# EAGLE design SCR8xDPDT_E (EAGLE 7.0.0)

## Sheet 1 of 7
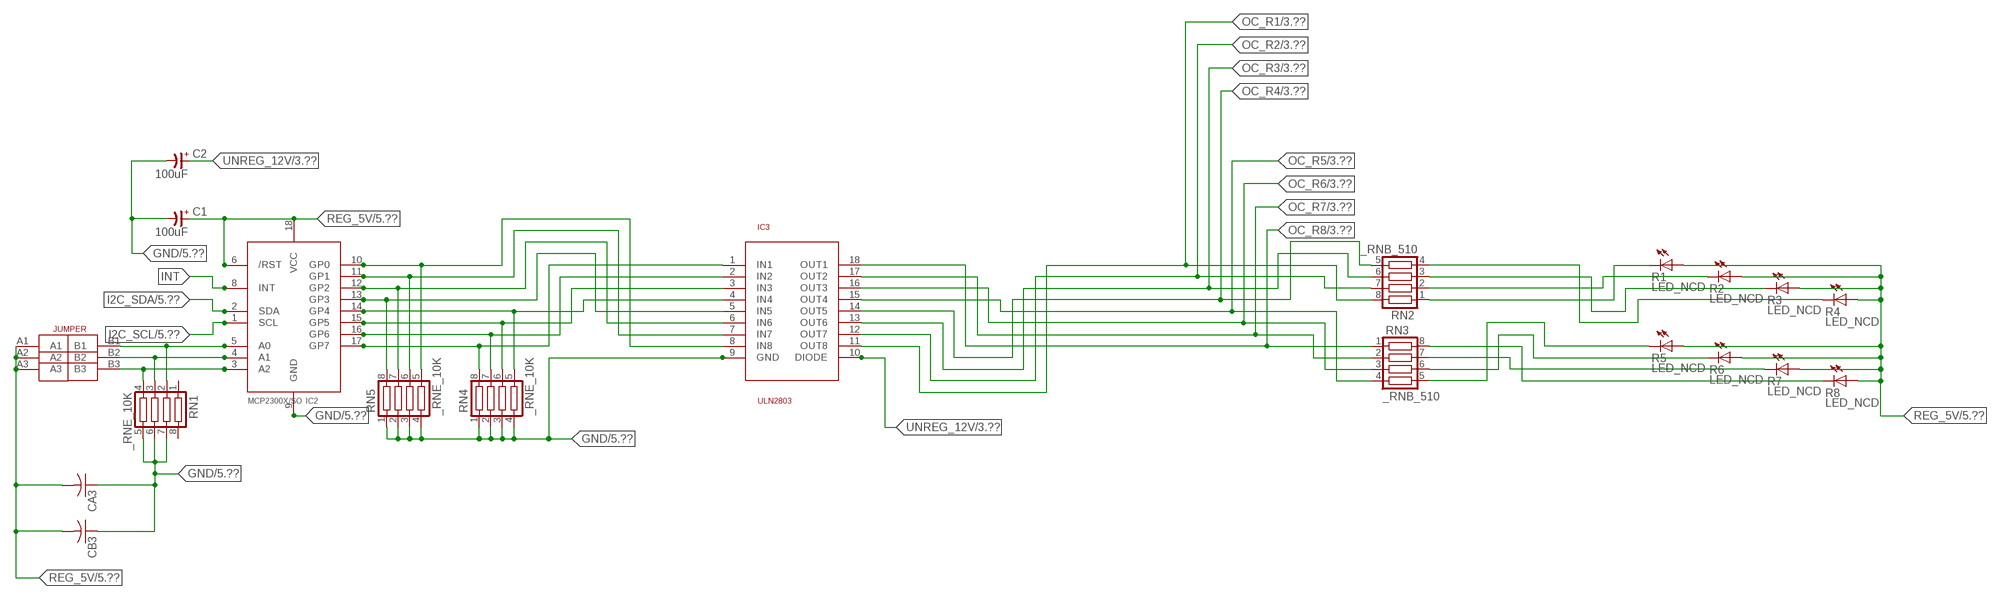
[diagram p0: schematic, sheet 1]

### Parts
C1  100uF  CP-E-025X060  [E-025X060]
C2  100uF  CP-E-025X060  [E-025X060]
CA3  CC1206KRX7R9BB104C1206K  [CC1206KRX7R9BB104]
CB3  TMK316F106ZL-TC1206K  [TMK316F106ZL-T]
IC2  MCP2300X/SO  [SO18W]
IC3  ULN2803  [SO18L]
R1  LED_NCD  [CHIPLED_0603]
R2  LED_NCD  [CHIPLED_0603]
R3  LED_NCD  [CHIPLED_0603]
R4  LED_NCD  [CHIPLED_0603]
R5  LED_NCD  [CHIPLED_0603]
R6  LED_NCD  [CHIPLED_0603]
R7  LED_NCD  [CHIPLED_0603]
R8  LED_NCD  [CHIPLED_0603]
RN1  _RNE_10K  [RNE]
RN2  _RNB_510  [RNB]
RN3  _RNB_510  [RNB]
RN4  _RNE_10K  [RNE]
RN5  _RNE_10K  [RNE]
U$18  JUMPER_3X2  [JUMPER_3X2]

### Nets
GND: C1.- C2.- CA3.1 CB3.1 IC2.9(GND) IC3.9(GND) RN1.5 RN1.6 RN1.7 RN4.1 RN4.2 RN4.3 RN4.4 RN5.1 RN5.2 RN5.3 RN5.4 ; also sheet 5,7
GP4: IC2.14(GP4) IC3.4(IN4) RN4.5
GP6: IC2.16(GP6) IC3.2(IN2) RN4.7
I2C_SCL: IC2.1(SCL) ; also sheet 5
I2C_SDA: IC2.2(SDA) ; also sheet 5
INT: IC2.8(INT)
N$6: IC2.5(A0) RN1.2 U$18.B1
N$7: IC2.4(A1) RN1.3 U$18.B2
N$8: IC2.3(A2) RN1.4 U$18.B3
N$20: R1.C RN2.1
N$21: IC2.12(GP2) IC3.6(IN6) RN5.7
N$22: IC2.11(GP1) IC3.7(IN7) RN5.6
N$23: IC2.10(GP0) IC3.8(IN8) RN5.5
N$29: R2.C RN2.2
N$30: R3.C RN2.3
N$31: R4.C RN2.4
N$32: R8.C RN3.8
N$81: R7.C RN3.7
N$82: R6.C RN3.6
N$83: R5.C RN3.5
N$89: IC2.13(GP3) IC3.5(IN5) RN5.8
N$93: IC2.15(GP5) IC3.3(IN3) RN4.6
N$94: IC2.17(GP7) IC3.1(IN1) RN4.8
OC_R1: IC3.11(OUT8) RN2.8 ; also sheet 3
OC_R2: IC3.12(OUT7) RN2.7 ; also sheet 3
OC_R3: IC3.13(OUT6) RN2.6 ; also sheet 3
OC_R4: IC3.14(OUT5) RN2.5 ; also sheet 3
OC_R5: IC3.15(OUT4) RN3.4 ; also sheet 3
OC_R6: IC3.16(OUT3) RN3.3 ; also sheet 3
OC_R7: IC3.17(OUT2) RN3.2 ; also sheet 3
OC_R8: IC3.18(OUT1) RN3.1 ; also sheet 3
REG_5V: C1.+ CA3.2 CB3.2 IC2.6(/RST) IC2.18(VCC) R1.A R2.A R3.A R4.A R5.A R6.A R7.A R8.A U$18.A1 U$18.A2 U$18.A3 ; also sheet 5,7
UNREG_12V: C2.+ IC3.10(DIODE) ; also sheet 3,5
Unconnected: RN1.1 RN1.8

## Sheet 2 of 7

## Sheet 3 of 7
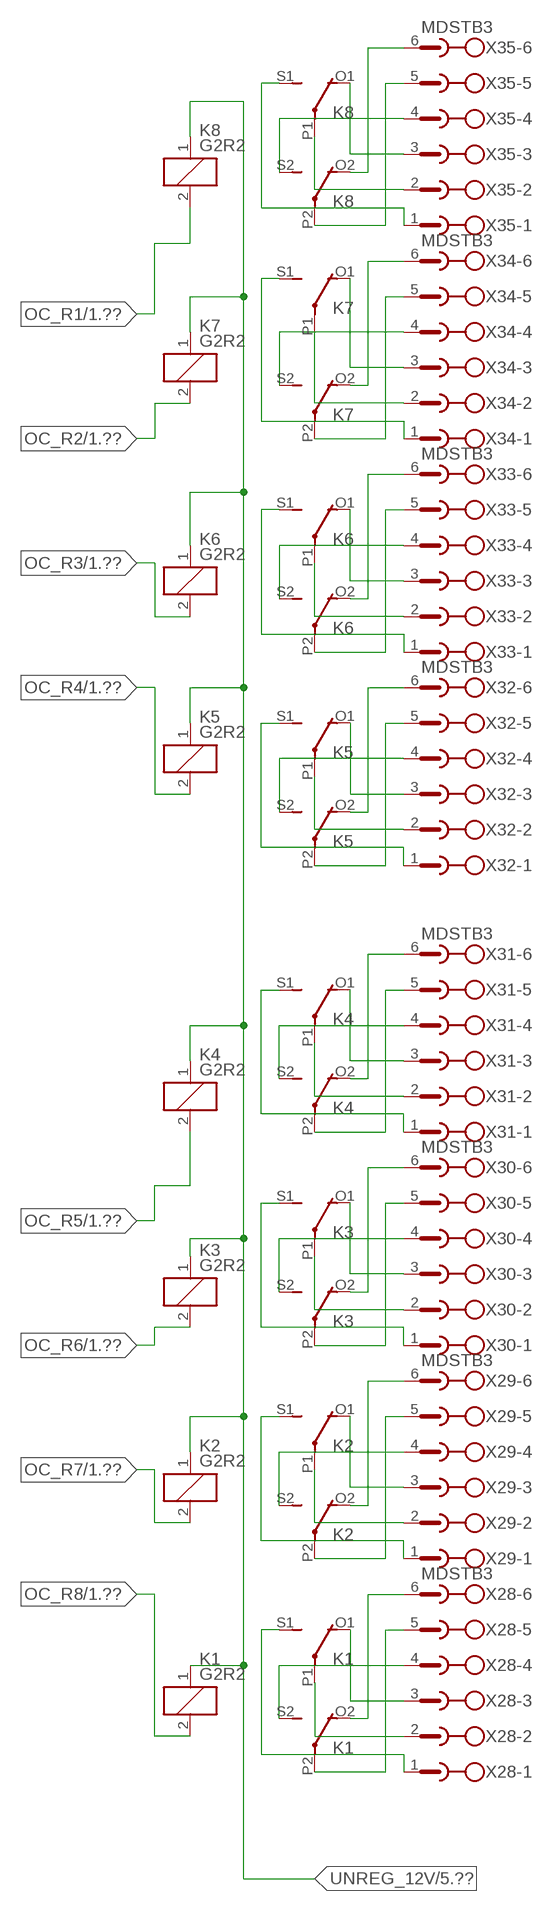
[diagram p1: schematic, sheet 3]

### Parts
K1  G2R2  [G2R2]
K2  G2R2  [G2R2]
K3  G2R2  [G2R2]
K4  G2R2  [G2R2]
K5  G2R2  [G2R2]
K6  G2R2  [G2R2]
K7  G2R2  [G2R2]
K8  G2R2  [G2R2]
X28  MDSTB3  [MDSTB3]
X29  MDSTB3  [MDSTB3]
X30  MDSTB3  [MDSTB3]
X31  MDSTB3  [MDSTB3]
X32  MDSTB3  [MDSTB3]
X33  MDSTB3  [MDSTB3]
X34  MDSTB3  [MDSTB3]
X35  MDSTB3  [MDSTB3]

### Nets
N$84: K1.P2(3:COM) X28.5
N$85: K1.O2(3:NC) X28.6
N$86: K1.S2(3:NO) X28.4
N$87: K1.P1(2:COM) X28.2
N$88: K1.O1(2:NC) X28.3
N$90: K1.S1(2:NO) X28.1
N$91: K2.P2(3:COM) X29.5
N$92: K2.O2(3:NC) X29.6
N$95: K2.S2(3:NO) X29.4
N$96: K2.S1(2:NO) X29.1
N$97: K2.P1(2:COM) X29.2
N$98: K2.O1(2:NC) X29.3
N$99: K3.P2(3:COM) X30.5
N$100: K3.O2(3:NC) X30.6
N$101: K4.P2(3:COM) X31.5
N$102: K4.O2(3:NC) X31.6
N$103: K3.S2(3:NO) X30.4
N$104: K4.S2(3:NO) X31.4
N$105: K3.O1(2:NC) X30.3
N$106: K4.O1(2:NC) X31.3
N$107: K4.P1(2:COM) X31.2
N$108: K3.P1(2:COM) X30.2
N$109: K3.S1(2:NO) X30.1
N$110: K4.S1(2:NO) X31.1
N$111: K5.O2(3:NC) X32.6
N$112: K5.P2(3:COM) X32.5
N$113: K5.S2(3:NO) X32.4
N$114: K5.P1(2:COM) X32.2
N$115: K5.S1(2:NO) X32.1
N$116: K5.O1(2:NC) X32.3
N$117: K6.P2(3:COM) X33.5
N$118: K6.O2(3:NC) X33.6
N$119: K6.P1(2:COM) X33.2
N$120: K6.S1(2:NO) X33.1
N$121: K7.P1(2:COM) X34.2
N$122: K8.P1(2:COM) X35.2
N$316: K8.P2(3:COM) X35.5
N$317: K8.O2(3:NC) X35.6
N$318: K6.O1(2:NC) X33.3
N$319: K8.O1(2:NC) X35.3
N$320: K7.O1(2:NC) X34.3
N$321: K7.O2(3:NC) X34.6
N$322: K7.P2(3:COM) X34.5
N$323: K6.S2(3:NO) X33.4
N$324: K7.S2(3:NO) X34.4
N$325: K7.S1(2:NO) X34.1
N$326: K8.S1(2:NO) X35.1
N$327: K8.S2(3:NO) X35.4
OC_R1: K8.2(1:C2) ; also sheet 1
OC_R2: K7.2(1:C2) ; also sheet 1
OC_R3: K6.2(1:C2) ; also sheet 1
OC_R4: K5.2(1:C2) ; also sheet 1
OC_R5: K4.2(1:C2) ; also sheet 1
OC_R6: K3.2(1:C2) ; also sheet 1
OC_R7: K2.2(1:C2) ; also sheet 1
OC_R8: K1.2(1:C2) ; also sheet 1
UNREG_12V: K1.1(1:C1) K2.1(1:C1) K3.1(1:C1) K4.1(1:C1) K5.1(1:C1) K6.1(1:C1) K7.1(1:C1) K8.1(1:C1) ; also sheet 1,5

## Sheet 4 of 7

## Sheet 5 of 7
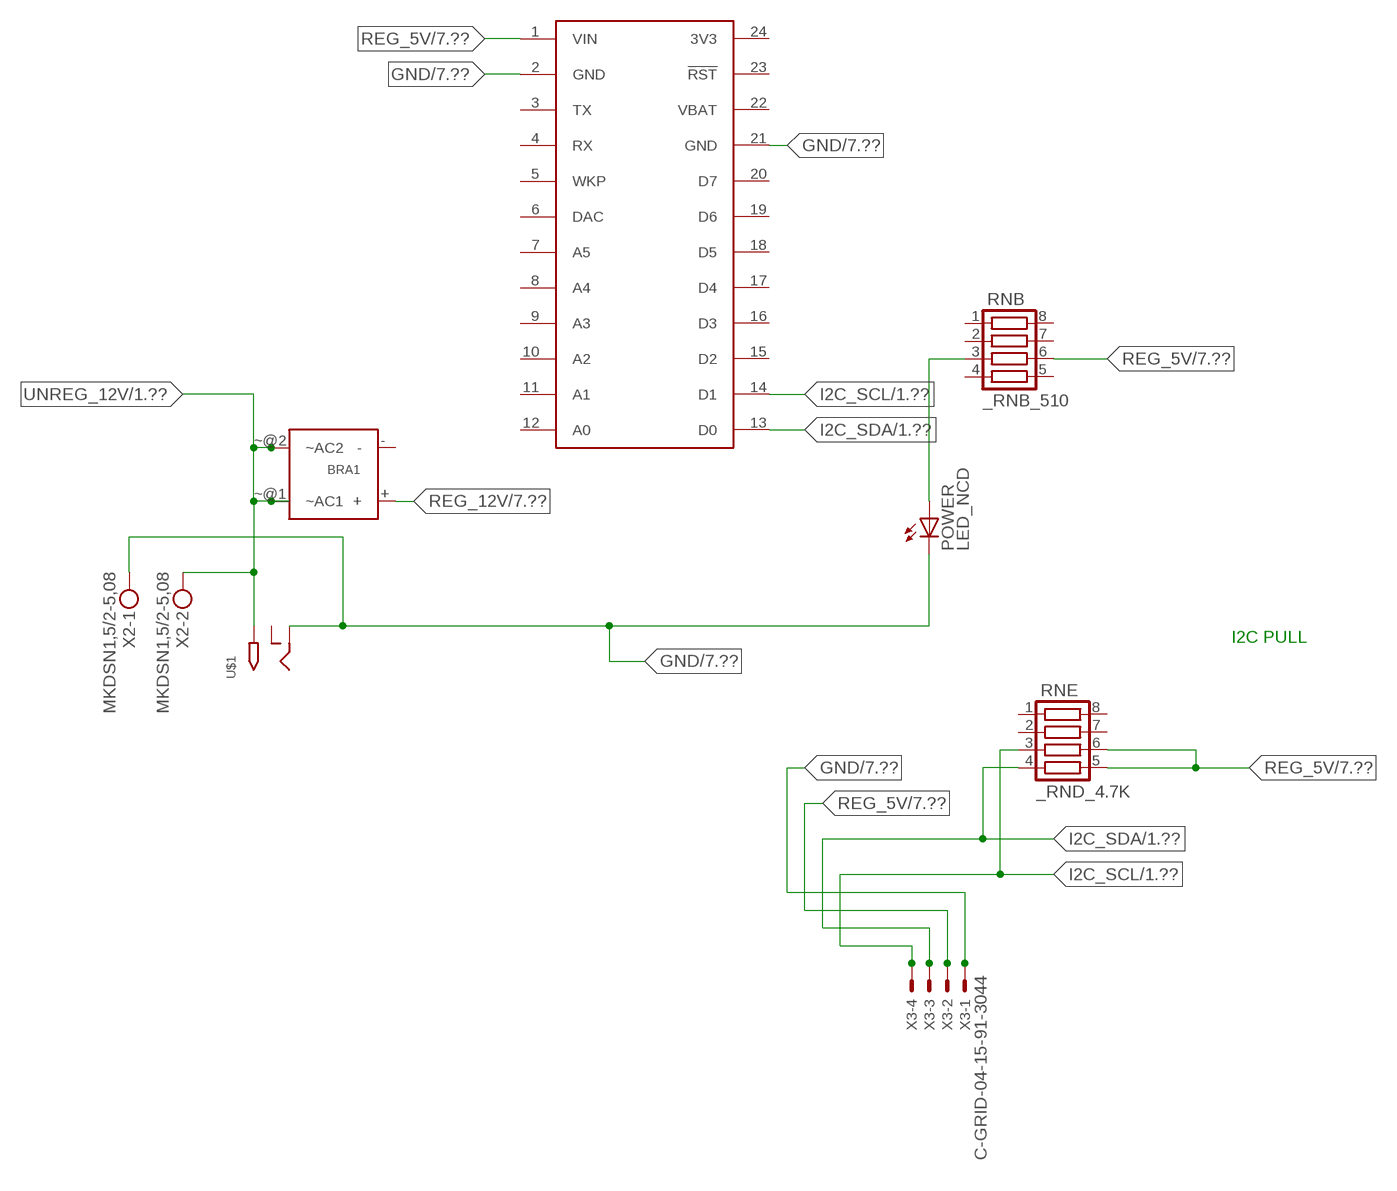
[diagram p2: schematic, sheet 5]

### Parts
BRA1  MB2S_  [MB2S]
POWER  LED_NCD  [CHIPLED_0603]
RNB  _RNB_510  [RNB]
RNE  _RND_4.7K  [RND]
S1  SPARK_CORECORE  [SPARK_CORE]
U$1  2.1MMJACK  [PJ-102A]
X2  MKDSN1,5/2-5,08  [MKDSN1,5/2-5,08]
X3  C-GRID-04-15-91-3044  [15-91-04]

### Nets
GND: POWER.C S1.2(GND) S1.21(GND) U$1.RING X2.1 X3.1 ; also sheet 1,7
I2C_SCL: RNE.3 S1.14(D1) X3.4 ; also sheet 1
I2C_SDA: RNE.4 S1.13(D0) X3.3 ; also sheet 1
N$2: POWER.A RNB.3
REG_5V: RNB.6 RNE.5 RNE.6 S1.1(VIN) X3.2 ; also sheet 1,7
REG_12V: BRA1.+ ; also sheet 7
UNREG_12V: BRA1.~@1(~AC1) BRA1.~@2(~AC2) U$1.TIP X2.2 ; also sheet 1,3
Unconnected: BRA1.- RNB.1 RNB.2 RNB.4 RNB.5 RNB.7 RNB.8 RNE.1 RNE.2 RNE.7 RNE.8 S1.3(TX) S1.4(RX) S1.5(WKP) S1.6(DAC) S1.7(A5) S1.8(A4) S1.9(A3) S1.10(A2) S1.11(A1) S1.12(A0) S1.15(D2) S1.16(D3) S1.17(D4) S1.18(D5) S1.19(D6) S1.20(D7) S1.23(!RST) U$1.RING_SW

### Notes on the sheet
- I2C PULL

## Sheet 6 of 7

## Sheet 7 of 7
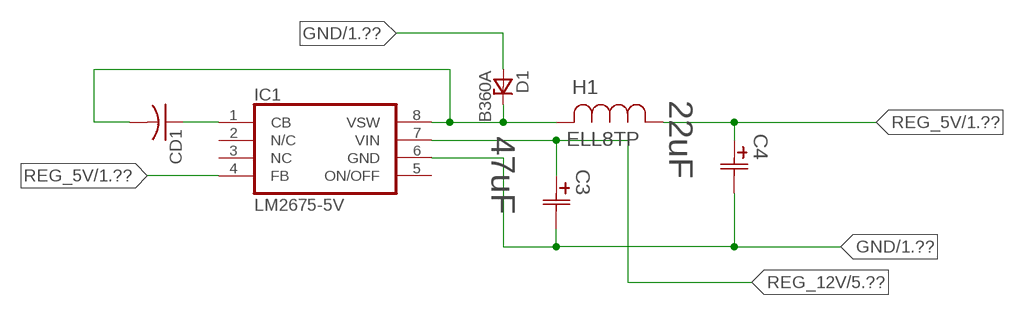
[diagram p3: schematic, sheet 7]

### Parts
C3  47uF  490-5463-6-NDCAP  [C2917(7343)-Y]
C4  22uF  490-5463-6-NDCAP  [C2917(7343)-Y]
CD1  _CD_10NF_50VC1206K  [_CD_10NF_50V]
D1  B360A  [DO214AC_ZENER]
H1  ELL8TP  [IND_ELL8TP]
IC1  LM2675-5V  LM2675  [SO-8]

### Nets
GND: C3.2(C2) C4.2(C2) D1.A IC1.6(GND) ; also sheet 1,5
N$1: CD1.2 D1.C H1.2 IC1.8(VSW)
N$3: CD1.1 IC1.1(CB)
REG_5V: C4.1(C1) H1.1 IC1.4(FB) ; also sheet 1,5
REG_12V: C3.1(C1) IC1.7(VIN) ; also sheet 5
Unconnected: IC1.2(N/C) IC1.5(ON/OFF)

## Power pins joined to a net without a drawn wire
3V3: S1.24(3V3)
NC: IC1.3(NC)
VBAT: S1.22(VBAT)

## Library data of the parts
BRA1 = NCD_ULTIMATE_LIBRARY:MB2S: Bridge Rectifier BRA MB2S 200V 500ma Digikey MB2S-TPMSTR-ND/MB2S-TP
C1 C2 = NCD_ULTIMATE_LIBRARY:CP-: Capacitors All Kinds POLARIZED CAP
C3 C4 = NCD_ULTIMATE_bhaskar:490-5463-6-ND: NCD CAP
CA3 = NCD_ULTIMATE_LIBRARY:CC1206KRX7R9BB104: Capacitor CA .1uF 50V SMT C1206K CC1206KRX7R9BB104
CB3 = NCD_ULTIMATE_LIBRARY:TMK316F106ZL-T: Capacitor CB 10uF SMT 1206 TMK316F106ZL-T
CD1 = NCD_ULTIMATE_LIBRARY:_CD_10NF_50V: Capacitor 10nF SMT
D1 = NCD_ULTIMATE_bhaskar:B360A: NCD DIODE B350A/B360A
H1 = NCD_ULTIMATE_bhaskar:ELL8TP: NCD coil
IC1 = NCD_ULTIMATE_bhaskar:LM2675: LM2675 NCD http://www.ti.com/lit/ds/symlink/lm2675.pdf
IC2 = NCD_ULTIMATE_LIBRARY:MCP2300X: Semiconductor Port Expander I/O 8-Bit I2C MCP23008 Inexpensive i2c i/o expander - 8 general purpose i/o pins with optional pullups
IC3 = NCD_ULTIMATE_LIBRARY:ULN2803: Semiconductor 8 O.C. N-Channel Transistor Driver Digikey ULN2803AFWGCELTR-ND/ULN2803AFWG,C,EL
K1-K8 = NCD_ULTIMATE_LIBRARY:G2R2: RELAY 2 x switch, Omron
POWER = NCD_ULTIMATE_bhaskar:LED_NCD
R1-R8 = NCD_ULTIMATE_LIBRARY:LED_NCD: LED Digikey 754-1132-2-ND/APT2012SRCPRV
RN1 RN4 RN5 = NCD_ULTIMATE_LIBRARY:_RNE_10K: Resistor Array RNE SMT 10K x 4 Single Resistor Source: http://www.ctscorp.com/components/Datasheets/CTSChipArrayDs.pdf Digikey 742C083103JPTR-ND/742C083103JP; OC_FARNELL: unknown; OC_NEWARK: unknown
RN2 RN3 RNB = NCD_ULTIMATE_LIBRARY:_RNB_510: Resistor Array RNB SMT 510 x 4 Single Resistor Source: http://www.ctscorp.com/components/Datasheets/CTSChipArrayDs.pdf Digikey 742C083511JPTR-ND/ 742C083511JP; OC_FARNELL: unknown; OC_NEWARK: unknown
RNE = NCD_ULTIMATE_LIBRARY:_RND_4.7K: Resistor Array RND SMT 4.7K x 4 Single Resistor Source: http://www.ctscorp.com/components/Datasheets/CTSChipArrayDs.pdf Digikey 742C083472JPTR-ND/742C083472JP; OC_FARNELL: unknown; OC_NEWARK: unknown
S1 = Spark:SPARK_CORE
U$1 = NCD_ULTIMATE_CONNECTORS:2.1MMJACK: 2.1mm x 5.5mm DC jack with internal switch. Digikey part #PJ-102A, 4UCON part #05537 By microbuilder.eu
U$18 = NCD_ULTIMATE_CONNECTORS:JUMPER_3X2
X2 = NCD_ULTIMATE_CONNECTORS:MKDSN1,5/2-5,08: MKDSN 1,5/ 2-5,08 Printklemme
X3 = NCD_ULTIMATE_CONNECTORS:C-GRID-04: CONNECTOR 4-Pos I2C wire to board 2.54 mm (0.100") pitch header Digikey WM1342-ND/0015912045; OC_FARNELL: unknown; OC_NEWARK: unknown
X28-X35 = NCD_ULTIMATE_LIBRARY:MDSTB3: PHOENIX

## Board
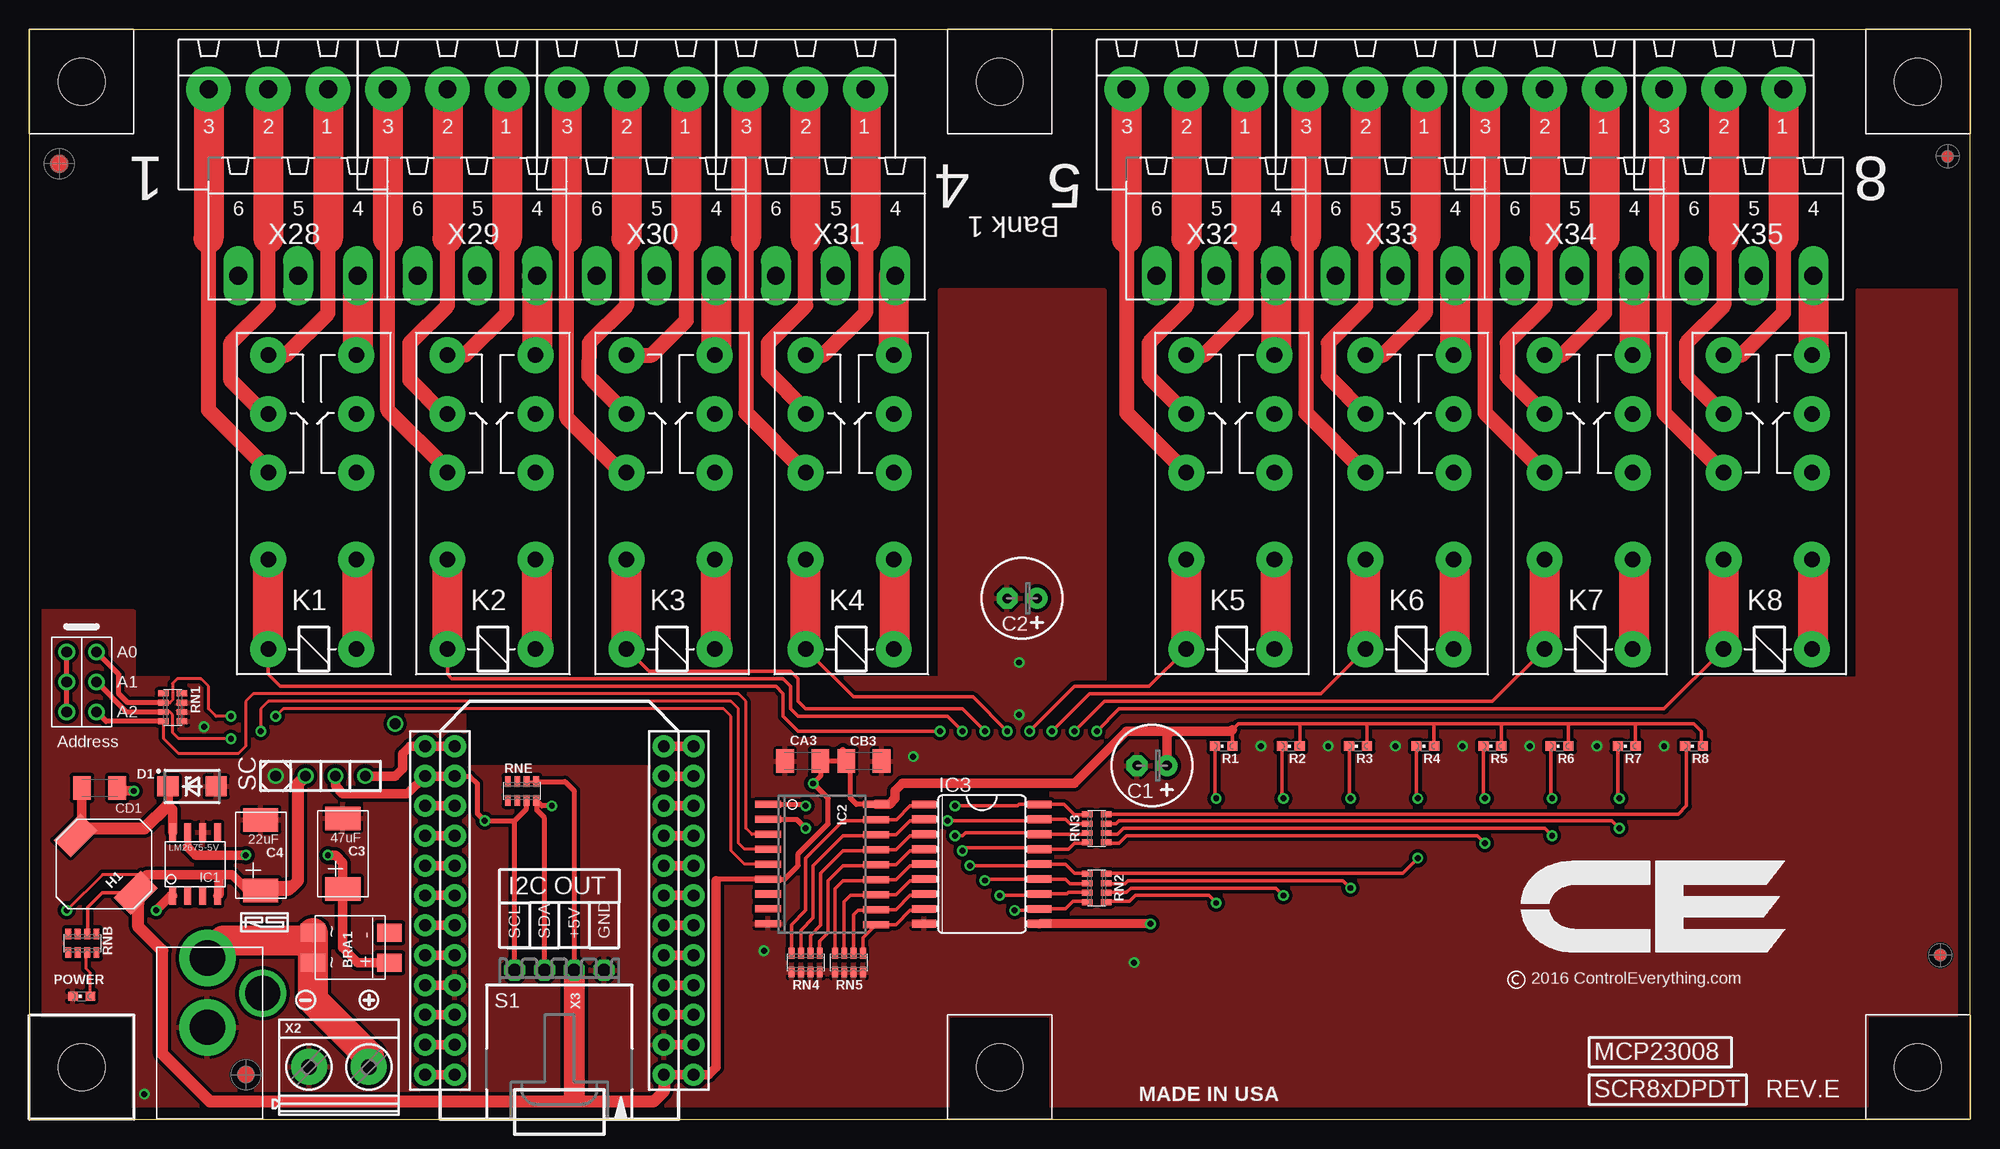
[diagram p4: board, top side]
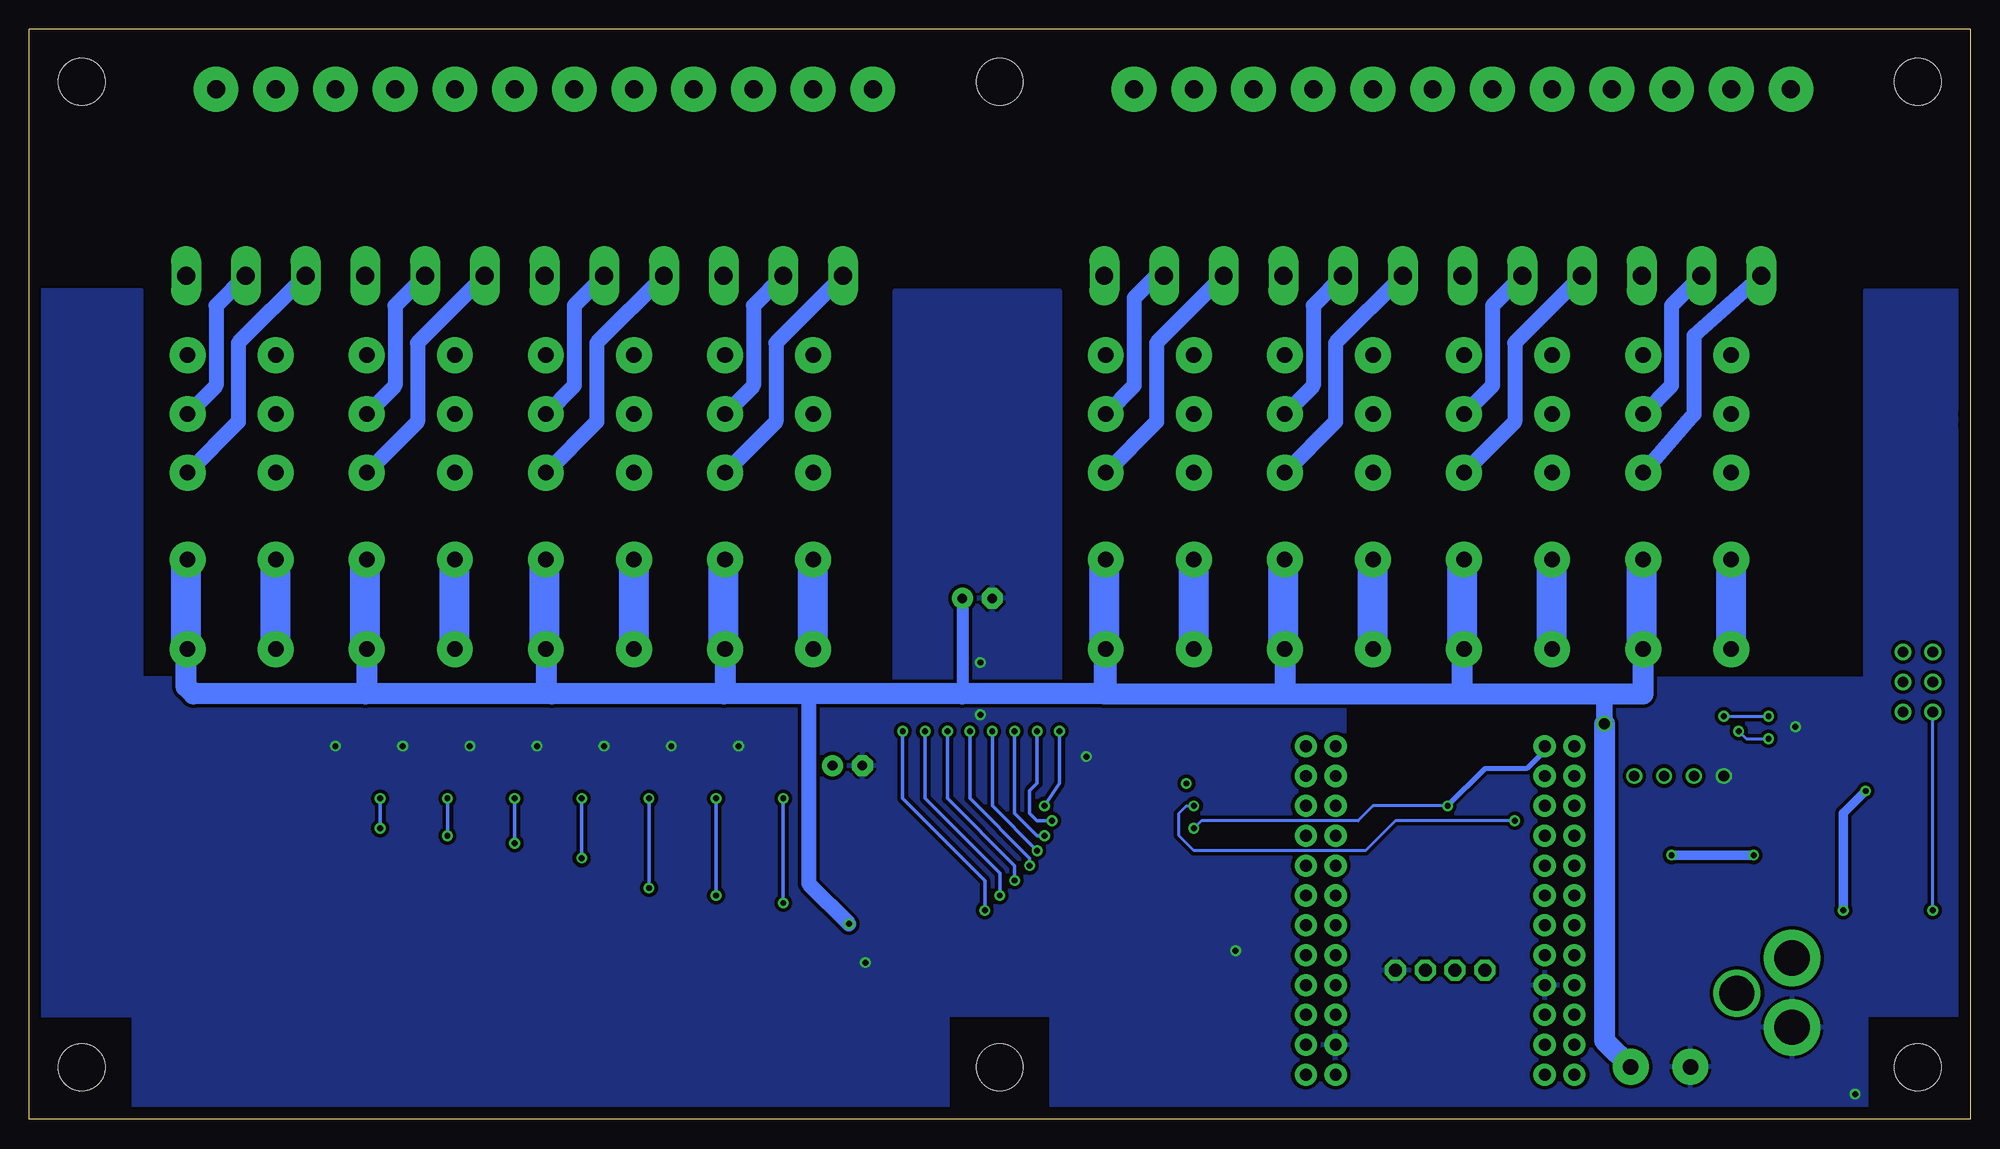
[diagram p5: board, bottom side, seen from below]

Size 165.1 x 92.71 mm. Coordinates in mm from the lower left corner, seen from the top.
Outline: 81.28,0 82.53,0
Outline: 0,59.99 0,59.05
Outline: 0,59.05 0,0 81.28,0
Outline: 81.28,0 165.1,0 165.1,92.71 0,92.71 0,59.05
Copper layers (1*16): Top 0.035mm / dielectric 1.5mm / Bottom 0.035mm
Design rules "default": minimum track width 10mil, minimum drill 24mil, track to track 8mil, track to pad 8mil, pad to pad 8mil, via to via 8mil, smd to smd 8mil, copper to edge 40mil, drill to drill 8mil, minimum pad ring 10mil, minimum via ring 8mil, stop-mask expansion 4mil, vias tented up to drill 0mil, thermal gap 10mil
Holes 3.96 mm at 4.45,4.45 4.45,4.45

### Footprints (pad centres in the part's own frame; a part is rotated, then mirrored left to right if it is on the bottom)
MB2S = smd 1.55 x 2.1: + 0,-6.5; - 2.54,-6.5; ~@1 0,0; ~@2 2.54,0
E-025X060 = drill 0.813 pad 1.778: + -1.27,0 | drill 0.813 pad 1.778 octagon: - 1.27,0
C2917(7343)-Y = smd 2 x 3: 1 -3,0; 2 3,0
CC1206KRX7R9BB104 = smd 1.5 x 2: 1 -1.5,0; 2 1.5,0
TMK316F106ZL-T = smd 1.5 x 2: 1 -1.5,0; 2 1.5,0
_CD_10NF_50V = smd 1.5 x 2: 1 -1.5,0; 2 1.5,0
DO214AC_ZENER = smd 1.8 x 1.7: A 2.05,0; C -2.05,0
IND_ELL8TP = smd 2.054 x 3.2 rotated 45: 1 -2.442,-2.696; 2 2.442,2.442
SO-8 = smd 0.6 x 1.55: 1 -1.905,-2.69; 2 -0.635,-2.69; 3 0.635,-2.69; 4 1.905,-2.69; 5 1.905,2.71; 6 0.635,2.71; 7 -0.635,2.71; 8 -1.905,2.71
SO18W = smd 0.6 x 2.2: 1 -4.445,-4.6; 2 -3.175,-4.6; 3 -1.905,-4.6; 4 -0.635,-4.6; 5 0.635,-4.6; 6 1.905,-4.6; 7 3.175,-4.6; 8 4.445,-4.6; 9 5.715,-4.6; 10 5.775,4.6; 11 4.505,4.6; 12 3.235,4.6; 13 1.965,4.6; 14 0.695,4.6; 15 -0.575,4.6; 16 -1.845,4.6; 17 -3.145,4.6; 18 -4.445,4.6
SO18L = smd 0.66 x 2.032: 1 -5.08,-4.902; 2 -3.81,-4.902; 3 -2.54,-4.902; 4 -1.27,-4.902; 5 0,-4.902; 6 1.27,-4.902; 7 2.54,-4.902; 8 3.81,-4.902; 9 5.08,-4.902; 10 5.08,4.902; 11 3.81,4.902; 12 2.54,4.902; 13 1.27,4.902; 14 0,4.902; 15 -1.27,4.902; 16 -2.54,4.902; 17 -3.81,4.902; 18 -5.08,4.902
G2R2 = drill 1.321 pad 3.048: 1 -2.54,-3.683; 2 -2.54,3.81; 3 5.08,-3.683; 4 5.08,3.81; O1 12.471,3.81; O2 12.471,-3.683; P1 17.45,3.81; P2 17.45,-3.683; S1 22.454,3.81; S2 22.454,-3.683
CHIPLED_0603 = smd 0.8 x 0.8: A 0,-0.75; C 0,0.75
CHIPLED_0603' = smd 0.8 x 0.876: A 0,-0.75; C 0,0.75
RNE = smd 0.5 x 0.9: 1 -1.2,-0.8; 2 -0.4,-0.8; 3 0.4,-0.8; 4 1.2,-0.8; 5 1.2,0.8; 6 0.4,0.8; 7 -0.4,0.8; 8 -1.2,0.8
RNB = smd 0.5 x 0.9: 1 -1.2,-0.8; 2 -0.4,-0.8; 3 0.4,-0.8; 4 1.2,-0.8; 5 1.2,0.8; 6 0.4,0.8; 7 -0.4,0.8; 8 -1.2,0.8
RND = smd 0.5 x 0.9: 1 -1.2,-0.8; 2 -0.4,-0.8; 3 0.4,-0.8; 4 1.2,-0.8; 5 1.2,0.8; 6 0.4,0.8; 7 -0.4,0.8; 8 -1.2,0.8
SPARK_CORE = drill 1.016 pad 1.88: 1 -8.89,13.97; 2 -8.89,11.43; 3 -8.89,8.89; 4 -8.89,6.35; 5 -8.89,3.81; 6 -8.89,1.27; 7 -8.89,-1.27; 8 -8.89,-3.81; 9 -8.89,-6.35; 10 -8.89,-8.89; 11 -8.89,-11.43; 12 -8.89,-13.97; 13 8.89,-13.97; 14 8.89,-11.43; 15 8.89,-8.89; 16 8.89,-6.35; 17 8.89,-3.81; 18 8.89,-1.27; 19 8.89,1.27; 20 8.89,3.81; 21 8.89,6.35; 22 8.89,8.89; 23 8.89,11.43; 24 8.89,13.97; 25 -11.43,13.97; 26 -11.43,11.43; 27 -11.43,8.89; 28 -11.43,6.35; 29 -11.43,3.81; 30 -11.43,1.27; 31 -11.43,-1.27; 32 -11.43,-3.81; 33 -11.43,-6.35; 34 -11.43,-8.89; 35 -11.43,-11.43; 36 -11.43,-13.97; 37 11.43,13.97; 38 11.43,11.43; 39 11.43,8.89; 40 11.43,6.35; 41 11.43,3.81; 42 11.43,1.27; 43 11.43,-1.27; 44 11.43,-3.81; 45 11.43,-6.35; 46 11.43,-8.89; 47 11.43,-11.43; 48 11.43,-13.97
PJ-102A = drill 3 pad 4.8: RING 0.1,-3.39; TIP 0.1,-9.29 | drill 3 pad 3.251: RING_SW -4.6,-6.29
PCB_MOUNTING_HOLE = hole 3.962: 4.445,4.445
JUMPER_3X2 = drill 0.9: A1 0,5.08; A2 0,2.54; A3 0,0; B1 2.54,5.08; B2 2.54,2.54; B3 2.54,0
MKDSN1,5/2-5,08 = drill 1.3 pad 3.048: 1 -2.561,0.025; 2 2.519,0.025
15-91-04 = drill 1.1 pad 1.778 octagon: 1 -3.81,-7.62; 2 -1.27,-7.62; 3 1.27,-7.62; 4 3.81,-7.62
MDSTB3 = drill 1.524 pad 3.81: 1 -3.81,-10.795; 2 1.27,-10.795; 3 6.35,-10.795 | drill 1.524 pad 2.54 long: 4 -6.35,5.08; 5 -1.27,5.08; 6 3.81,5.08

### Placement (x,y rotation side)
BRA1  24.13,13.34 90 top
C1  95.5,30.1 180 top
C2  84.45,44.32 180 top
C3  26.67,22.61 90 top
C4  19.68,22.48 90 top
CA3  65.79,30.48 0 top
CB3  70.99,30.48 180 top
CD1  5.97,28.19 180 top
D1  13.84,28.32 0 top
H1  6.35,21.72 90 top
IC1  14.1,21.72 0 top
IC2  67.44,22.35 270 top
IC3  81.03,21.72 270 top
K1  24.13,42.54 90 top
K2  39.37,42.54 90 top
K3  54.61,42.54 90 top
K4  69.85,42.54 90 top
K5  102.23,42.54 90 top
K6  117.47,42.54 90 top
K7  132.72,42.54 90 top
K8  147.96,42.54 90 top
POWER  4.45,10.48 90 top
R1  LED_NCD  [CHIPLED_0603']  101.6,31.75 90 top
R2  LED_NCD  [CHIPLED_0603']  107.31,31.75 90 top
R3  LED_NCD  [CHIPLED_0603']  113.03,31.75 90 top
R4  LED_NCD  [CHIPLED_0603']  118.75,31.75 90 top
R5  LED_NCD  [CHIPLED_0603']  124.46,31.75 90 top
R6  LED_NCD  [CHIPLED_0603']  130.18,31.75 90 top
R7  LED_NCD  [CHIPLED_0603']  135.89,31.75 90 top
R8  LED_NCD  [CHIPLED_0603']  141.6,31.75 90 top
RN1  12.19,35.05 270 top
RN2  90.81,19.69 90 top
RN3  90.81,24.77 270 top
RN4  66.04,13.34 0 top
RN5  69.72,13.34 0 top
RNB  4.51,14.99 0 top
RNE  41.91,27.94 0 top
S1  45.09,17.78 180 top
U$1  15.24,4.45 180 top
U$4  [VISION_REF10]  162.56,13.97 270 top
U$6  PCB_MOUNTING_HOLE  [PCB_MOUNTING_HOLE]  87,0 90 top
U$9  PCB_MOUNTING_HOLE  [PCB_MOUNTING_HOLE]  87,83.82 90 top
U$10  [VISION_REF15]  18.41,3.81 0 top
U$11  PCB_MOUNTING_HOLE  [PCB_MOUNTING_HOLE]  165.1,0 90 top
U$13  PCB_MOUNTING_HOLE  [PCB_MOUNTING_HOLE]  8.89,83.82 90 top
U$14  PCB_MOUNTING_HOLE  [PCB_MOUNTING_HOLE]  165.1,83.82 90 top
U$16  [VISION_REF10]  163.19,81.91 270 top
U$17  [VISION_REF15]  2.54,81.28 270 top
U$18  3.17,34.67 0 top
U$21  [ICON_USA]  94.36,1.52 0 top
U$22  [ICON_MINUS]  23.5,10.16 180 top
U$24  [ICON_PLUS]  28.89,10.16 90 top
X2  26.35,4.45 0 top
X3  45.09,5.08 180 top
X28  21.59,76.83 180 top
X29  36.83,76.83 180 top
X30  52.07,76.83 180 top
X31  67.31,76.83 180 top
X32  99.69,76.83 180 top
X33  114.94,76.83 180 top
X34  130.18,76.83 180 top
X35  145.41,76.83 180 top

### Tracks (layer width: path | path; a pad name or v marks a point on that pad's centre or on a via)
GND  (via drill 0.5, 0.9)
  other vias: 14.86,33.4 62.48,14.35 127.64,31.75 93.98,13.34 133.35,31.75 139.06,31.75 121.92,31.75 116.2,31.75 110.49,31.75 104.78,31.75 75.18,30.86 84.2,34.42 84.2,38.86 9.78,2.16 20.95,29.21
  pour Bottom (isolate 0.305): -1.27,8.89 8.89,8.89 8.89,0 78.11,0 78.11,8.89 91.44,8.89 91.44,70.48 77.47,70.48 77.47,37.46 8.89,37.46 8.89,70.48 -1.27,70.48
  pour Top (isolate 0.305): -3.17,8.89 8.89,8.89 8.89,0 78.11,0 78.11,8.89 91.44,8.89 91.44,70.48 77.47,70.48 77.47,37.46 8.89,37.46 8.89,43.18 -3.17,43.18
  pour Top (isolate 0.305): 87,37.46 155.57,37.46 155.57,70.48 168.28,70.48 168.28,8.89 156.21,8.89 156.21,0 87,0
  pour Bottom (isolate 0.305): 87,0 87,37.46 155.57,37.46 155.57,70.48 170.81,70.48 170.81,8.89 156.21,8.89 156.21,0
GP4
  Top 0.305: RN4.5 67.24,15.17 67.94,15.88 67.94,20.32 69.22,21.59 71.97,21.59 IC2.14 73.73,21.66 74.93,22.86 76,22.86 IC3.4
GP6
  Top 0.305: RN4.7 65.64,16.11 66.67,17.14 66.67,21.59 69.22,24.13 71.97,24.13 IC2.16 73.73,24.2 74.93,25.4 76,25.4 IC3.2
I2C_SCL  (via drill 0.5, 0.9)
  Top 0.406: IC2.1 65.91,26.8 v66.04,26.67 | X3.4 41.27,25.4 | 41.27,25.4 42.29,26.42 42.29,27.12 RNE.3 | S1.14 37.47,29.21 38.1,28.57 38.1,26.04 v38.73,25.4 41.27,25.4
  Top 0.813: v26.04,29.21 26.04,28.32 26.67,27.69 32.13,27.69 33.66,29.21
  Bottom 0.254: v38.73,25.4 48.9,25.4 51.44,22.86 66.04,22.86 67.31,24.13 67.31,26.04 66.67,26.67 v66.04,26.67
I2C_SDA  (via drill 0.5, 0.9)
  Top 0.406: IC2.2 65.28,25.53 v66.04,24.77 | X3.3 43.81,25.65 43.18,26.29 43.18,27.07 RNE.4 43.58,26.67 v44.45,26.67
  Top 0.813: v28.57,29.21 31.11,29.21 31.75,29.85 31.75,31.12 32.38,31.75 33.66,31.75
  Bottom 0.254: v44.45,26.67 50.8,26.67 52.07,25.4 65.41,25.4 v66.04,24.77
  Bottom 0.406: S1.13 36.2,31.37 37.72,29.85 41.27,29.85 v44.45,26.67
N$1
  Top 0.813: H1.2 3.88,24.77 | D1.C 11.79,26.78 12.19,26.38 IC1.8 | CD1.2 4.47,24.79 4.45,24.77
  Top 1.016: 3.88,24.77 4.45,24.77 9.78,24.77 11.79,26.78
N$2
  Top 0.254: POWER.A 5.2,12.46 4.83,12.83 4.83,14.1 RNB.3
  Top 0.406: 4.95,14.14 RNB.3
N$3  (via drill 0.5)
  Top 0.813: IC1.1 12.04,19.03 v10.79,17.78 | v8.89,27.94 7.72,27.94 CD1.1
  Bottom 0.813: v10.79,17.78 10.79,26.04 v8.89,27.94
N$6  (via drill 0.5)
  Top 0.254: IC2.5 60.83,21.72 59.69,22.86 59.69,34.29 59.05,34.92 21.59,34.92 v20.95,34.29 | v17.14,34.29 15.88,34.29 15.24,34.92 15.24,36.83 14.61,37.46 12.57,37.46 12.19,37.08 12.19,35.69 11.94,35.43 11.41,35.43 RN1.2
  Top 0.406: RN1.2 8.36,35.45 7.62,36.2 7.62,37.85 U$18.B1
  Bottom 0.254: v20.95,34.29 v17.14,34.29
N$7  (via drill 0.5)
  Top 0.254: IC2.4 60.83,22.99 60.33,23.5 60.33,34.92 59.69,35.56 20.32,35.56 19.68,34.92 v19.68,33.02 | v17.14,32.38 12.7,32.38 12.19,32.89 12.19,34.42 11.94,34.67 11.41,34.67 RN1.3
  Top 0.406: RN1.3 8.27,34.65 U$18.B2
  Bottom 0.254: v19.68,33.02 19.05,32.38 v17.14,32.38
N$8
  Top 0.254: IC2.3 61.47,24.26 60.96,24.77 60.96,35.56 60.33,36.2 19.05,36.2 18.41,35.56 18.41,31.75 17.78,31.12 12.7,31.12 11.43,32.38 11.43,33.81 RN1.4
  Top 0.406: RN1.4 6.53,33.85 U$18.B3
N$20  (via drill 0.5)
  Top 0.305: R1.C 100.85,27.42 v100.97,27.3 | v100.97,18.41 100.33,19.05 94.11,19.05 93.6,18.54 91.66,18.54 RN2.1
  Bottom 0.305: v100.97,27.3 v100.97,18.41
N$21
  Top 0.305: RN5.7 69.32,18.52 69.85,19.05 71.97,19.05 IC2.12 73.73,19.12 74.93,20.32 76,20.32 IC3.6
N$22
  Top 0.305: RN5.6 70.12,17.42 70.48,17.78 71.97,17.78 IC2.11 73.73,17.85 74.93,19.05 76,19.05 IC3.7
N$23
  Top 0.254: 71.97,16.51 IC2.10
  Top 0.305: RN5.5 70.92,15.46 IC2.10 73.73,16.58 74.93,17.78 76,17.78 IC3.8
N$29  (via drill 0.5)
  Top 0.305: R2.C 106.56,27.42 v106.68,27.3 | v106.68,19.05 106.05,19.69 93.73,19.69 93.34,19.3 91.62,19.3 RN2.2
  Bottom 0.305: v106.68,27.3 v106.68,19.05
N$30  (via drill 0.5)
  Top 0.305: R3.C 112.28,27.42 v112.39,27.3 | v112.39,19.69 111.76,20.32 93.47,20.32 93.22,20.07 91.62,20.07 RN2.3
  Bottom 0.305: v112.39,27.3 v112.39,19.69
N$31  (via drill 0.5)
  Top 0.305: R4.C 118,27.42 v118.11,27.3 | v118.11,22.23 116.84,20.96 91.67,20.96 RN2.4
  Bottom 0.305: v118.11,27.3 v118.11,22.23
N$32
  Top 0.305: RN3.8 140.26,25.96 140.97,26.67 140.97,31.64 R8.C
N$81  (via drill 0.5)
  Top 0.305: R7.C 135.14,27.42 v135.25,27.3 | v135.25,24.77 134.62,25.4 92.71,25.4 92.46,25.15 91.62,25.15 RN3.7
  Bottom 0.305: v135.25,27.3 v135.25,24.77
N$82  (via drill 0.5)
  Top 0.305: R6.C 129.43,27.42 v129.54,27.3 | v129.54,24.13 128.91,24.77 93.09,24.77 92.58,24.26 91.71,24.26 RN3.6
  Bottom 0.305: v129.54,27.3 v129.54,24.13
N$83  (via drill 0.5)
  Top 0.305: R5.C 123.71,27.42 v123.83,27.3 | v123.83,23.5 123.19,24.13 93.34,24.13 92.71,23.5 91.67,23.5 RN3.5
  Bottom 0.305: v123.83,27.3 v123.83,23.5
N$84
  Bottom 1.27: X28.5 25.4,69.22 25.4,62.41 K1.P2
N$85
  Bottom 1.27: X28.6 23.5,66.67 23.5,59.97 K1.O2
N$86
  Top 2.54: X28.4 27.94,65.13 K1.S2
N$87
  Top 1.27: K1.P1 20.02,59.99 17.14,62.86 17.14,66.04 20.32,69.22 20.32,74.93
  Top 2.54: X28.2 20.32,74.93
N$88
  Top 1.27: K1.O1 20.32,55.24 15.24,60.32 15.24,74.93
  Top 2.54: X28.3 15.24,74.93
N$89
  Top 0.305: RN5.8 68.52,19.63 69.22,20.32 71.97,20.32 IC2.13 73.73,20.39 74.93,21.59 76,21.59 IC3.5
N$90
  Top 1.27: K1.S1 21.82,65 25.4,68.58 25.4,74.93
  Top 2.54: X28.1 25.4,74.93
N$91
  Bottom 1.27: X29.5 40.64,69.22 40.64,62.41 K2.P2
N$92
  Bottom 1.27: X29.6 38.73,66.04 38.73,59.33 K2.O2
N$93
  Top 0.305: RN4.6 66.44,15.64 67.31,16.51 67.31,20.96 69.22,22.86 71.97,22.86 IC2.15 73.73,22.93 74.93,24.13 76,24.13 IC3.3
N$94
  Top 0.305: RN4.8 64.84,16.58 66.04,17.78 66.04,22.23 69.22,25.4 71.94,25.4 IC2.17 73.76,25.5 74.93,26.67 76,26.67 IC3.1
N$95
  Top 2.54: X29.4 43.18,65.13 K2.S2
N$96
  Top 1.27: K2.S1 37.08,65.02 40.64,68.58 40.64,74.93
  Top 2.54: X29.1 40.64,74.93
N$97
  Top 1.27: K2.P1 35.26,59.99 32.38,62.86 32.38,66.04 35.56,69.22 35.56,74.93
  Top 2.54: X29.2 35.56,74.93
N$98
  Top 1.27: K2.O1 35.56,55.24 30.48,60.32 30.48,74.93
  Top 2.54: X29.3 30.48,74.93
N$99
  Bottom 1.27: X30.5 55.88,69.22 55.88,62.41 K3.P2
N$100
  Bottom 1.27: X30.6 53.98,66.04 53.98,59.33 K3.O2
N$101
  Bottom 1.27: X31.5 69.22,71.75 71.12,69.85 71.12,62.41 K4.P2
N$102
  Bottom 1.27: X31.6 69.22,66.04 69.22,59.33 K4.O2
N$103
  Top 2.54: X30.4 58.42,65.13 K3.S2
N$104
  Top 2.54: X31.4 73.53,71.75 K4.S2
N$105
  Top 1.27: K3.O1 50.39,55.02 45.72,59.69 45.72,74.93
  Top 2.54: X30.3 45.72,74.93
N$106
  Top 1.27: 60.96,74.93 60.96,60.1 K4.O1
  Top 2.54: X31.3 60.96,74.93
N$107
  Top 1.27: K4.P1 66.04,60.32 62.87,63.5 62.87,66.04 66.04,69.22 66.04,74.93
  Top 2.54: 66.04,74.93 X31.2
N$108
  Top 1.27: 50.8,74.93 50.8,69.22 47.62,66.04 47.57,63.25 47.93,62.86 K3.P1
  Top 2.54: X30.2 50.8,74.93
N$109
  Top 1.27: 55.88,74.93 55.88,67.94 52.93,65 K3.S1
  Top 2.54: X30.1 55.88,74.93
N$110
  Top 1.27: 71.12,74.93 71.12,68.58 67.54,65 K4.S1
  Top 2.54: X31.1 71.12,74.93
N$111
  Bottom 1.27: X32.6 101.6,66.04 101.6,59.33 K5.O2
N$112
  Bottom 1.27: X32.5 103.5,69.22 103.5,62.41 K5.P2
N$113
  Top 2.54: X32.4 106.05,65.13 K5.S2
N$114
  Top 1.27: 98.42,74.93 98.42,69.22 95.25,66.04 95.25,63.17 K5.P1
  Top 2.54: X32.2 98.42,74.93
N$115
  Top 1.27: 103.5,74.93 103.5,68.58 99.92,65 K5.S1
  Top 2.54: X32.1 103.5,74.93
N$116
  Top 1.27: 93.34,74.93 93.34,60.1 K5.O1
  Top 2.54: X32.3 93.34,74.93
N$117
  Bottom 1.27: X33.5 118.75,69.22 118.75,62.41 K6.P2
N$118
  Bottom 1.27: X33.6 116.84,66.04 116.84,59.33 K6.O2
N$119
  Top 1.27: 113.67,74.93 113.67,69.22 110.49,66.04 110.49,63.17 K6.P1
  Top 2.54: X33.2 113.67,74.93
N$120
  Top 1.27: 118.75,74.93 118.75,68.58 115.16,65 K6.S1
  Top 2.54: X33.1 118.75,74.93
N$121
  Top 1.27: 128.91,74.93 128.91,69.22 125.73,66.04 125.73,63.17 K7.P1
  Top 2.54: X34.2 128.91,74.93
N$122
  Top 1.27: 144.15,74.93 144.15,69.22 140.97,66.04 140.97,63.17 K8.P1
  Top 2.54: X35.2 144.15,74.93
N$316
  Bottom 1.27: X35.5 149.22,69.22 149.22,62.41 K8.P2
N$317
  Bottom 1.27: X35.6 147.32,66.04 147.32,59.33 K8.O2
N$318
  Top 1.27: 108.58,74.93 108.58,60.1 K6.O1
  Top 2.54: X33.3 108.58,74.93
N$319
  Top 1.27: 139.06,74.93 139.06,60.1 K8.O1
  Top 2.54: X35.3 139.06,74.93
N$320
  Top 1.27: 123.83,74.93 123.83,60.1 K7.O1
  Top 2.54: X34.3 123.83,74.93
N$321
  Bottom 1.27: X34.6 132.08,66.04 132.08,59.33 K7.O2
N$322
  Bottom 1.27: X34.5 133.99,69.22 133.99,62.41 K7.P2
N$323
  Top 2.54: X33.4 121.28,65.13 K6.S2
N$324
  Top 2.54: X34.4 136.53,65.13 K7.S2
N$325
  Top 1.27: 133.99,74.93 133.99,68.58 130.4,65 K7.S1
  Top 2.54: X34.1 133.99,74.93
N$326
  Top 1.27: 149.22,74.93 149.22,68.58 145.64,65 K8.S1
  Top 2.54: X35.1 149.22,74.93
N$327
  Top 2.54: X35.4 151.76,65.13 K8.S2
OC_R1  (via drill 0.5)
  Top 0.305: RN2.8 89.95,18.54 88.77,18.54 88.14,17.91 IC3.11 85.8,17.78 v83.82,17.78 | K8.2 139.06,34.92 92.71,34.92 v90.81,33.02
  Bottom 0.305: v90.81,33.02 90.81,27.3 83.82,20.32 v83.82,17.78
OC_R2  (via drill 0.5)
  Top 0.305: RN2.7 89.99,19.3 88.39,19.3 88.27,19.18 IC3.12 85.8,19.05 v82.55,19.05 | v88.9,33.02 91.44,35.56 124.46,35.56 K7.2
  Bottom 0.305: v88.9,33.02 88.9,27.3 82.55,20.96 v82.55,19.05
OC_R3  (via drill 0.5)
  Top 0.305: RN2.6 89.99,20.07 88.52,20.07 88.14,20.45 IC3.13 81.53,20.45 81.41,20.32 v81.28,20.32 | K6.2 109.86,36.2 90.17,36.2 v87,33.02
  Bottom 0.305: v87,33.02 87,27.3 81.28,21.59 v81.28,20.32
OC_R4  (via drill 0.5)
  Top 0.305: RN2.5 89.94,20.96 88.9,20.96 88.14,21.72 IC3.14 85.8,21.59 v80.01,21.59 | v85.09,33.02 88.9,36.83 95.25,36.83 K5.2
  Bottom 0.305: v85.09,33.02 85.09,27.3 80.01,22.23 v80.01,21.59
OC_R5  (via drill 0.5)
  Top 0.305: RN3.4 89.94,23.5 88.9,23.5 88.39,22.99 IC3.15 85.8,23.11 79.63,23.11 v79.38,22.86 | v83.19,33.02 80.26,35.94 70.1,35.94 K4.2
  Bottom 0.305: v83.19,33.02 83.19,26.67 v79.38,22.86
OC_R6  (via drill 0.5)
  Top 0.305: RN3.3 89.9,24.26 IC3.16 85.8,24.38 79.63,24.38 79.38,24.13 v78.74,24.13 | v81.28,33.02 79.38,34.92 66.04,34.92 65.41,35.56 65.41,37.46 64.77,38.1 52.7,38.1 K3.2
  Bottom 0.305: v81.28,33.02 81.28,26.04 79.38,24.13 v78.74,24.13
OC_R7  (via drill 0.5)
  Top 0.305: RN3.2 89.99,25.15 88.52,25.15 88.14,25.53 IC3.17 85.8,25.4 v78.11,25.4 | v79.38,33.02 78.11,34.29 65.41,34.29 64.77,34.92 64.77,36.83 64.14,37.46 35.94,37.46 35.56,37.85 K2.2
  Bottom 0.305: v79.38,33.02 79.38,28.57 80.01,27.94 80.01,26.04 79.38,25.4 v78.11,25.4
OC_R8  (via drill 0.5)
  Top 0.305: RN3.1 89.95,25.91 88.9,25.91 88.01,26.8 IC3.18 84.2,26.8 84.07,26.67 v78.74,26.67 | v77.47,33.02 65.41,33.02 64.14,34.29 64.14,36.2 63.5,36.83 21.34,36.83 20.32,37.85 K1.2
  Bottom 0.305: v77.47,33.02 77.47,28.57 v78.74,26.67
REG_5V  (via drill 0.5, 0.9)
  Top 0.254: RNE.6 RNE.5 | 9.96,20.83 6.22,20.83 v3.17,17.78
  Top 0.305: R1.A 102.35,33.13 102.87,33.66 107.95,33.66 | 107.95,33.66 113.67,33.66 | 113.67,33.66 119.38,33.66 | 119.38,33.66 125.09,33.66 | 125.09,33.66 130.81,33.66 | 130.81,33.66 136.53,33.66 | 136.53,33.66 141.6,33.66 142.24,33.02 142.24,31.87 R8.A | R7.A 136.64,33.54 136.53,33.66 | R6.A 130.93,33.54 130.81,33.66 | R5.A 125.21,33.54 125.09,33.66 | R4.A 119.5,33.54 119.38,33.66 | R3.A 113.78,33.54 113.67,33.66 | R2.A 108.06,33.54 107.95,33.66 | H1.1 6.19,19.28 4.95,18.03 4.95,15.83 RNB.6
  Top 0.406: U$18.A3 U$18.A2 U$18.A1 | IC2.18 70.36,26.8 69.85,27.3 69.85,30.76 CB3.2 CA3.2 67.29,29.19 v66.67,28.57 67.94,27.3 67.94,25.15 65.41,22.61 65.41,21.59 64.26,20.45 IC2.6 | 62.71,20.32 IC2.6 | RNE.5 45.55,28.74 46.35,27.94 X3.2 | IC2.6 58.55,20.45 58.42,20.32
  Top 0.61: 69.22,31.39 CB3.2
  Top 0.813: IC2.18 73.15,26.8 73.66,27.3 73.66,27.94 74.3,28.57 88.9,28.57 93.34,33.02 97.16,33.02 | 97.16,33.02 102.23,33.02 102.35,33.13 | C1.+ 96.77,32.64 97.16,33.02 | 16.13,20.83 9.96,20.83 H1.1 | 16.13,20.83 17.27,20.83 18.41,19.69 20.75,19.69 C4.1 | IC1.4 16.13,19.15 16.13,20.83 | S1.1 57.78,3.81 58.42,4.45 58.42,20.32
  Top 1.016: 46.35,2.16 46.35,1.52 | 46.35,1.52 15.37,1.52 11.3,5.59 11.3,14.35 9.27,16.38 9.27,18.41 H1.1 | 22.05,19.69 22.23,19.69 22.86,20.32 22.86,28.57 v23.5,29.21 | S1.1 53.98,2.41 53.09,1.52 46.35,1.52
  Top 1.27: 20.75,19.69 22.05,19.69
  Top 1.778: X3.2 46.35,2.16
  Bottom 0.254: v3.17,17.78 U$18.A3
REG_12V  (via drill 0.5)
  Top 0.61: IC1.7 13.46,23.16 | 14.1,22.48 14.15,22.48
  Top 0.813: v18.41,22.48 14.15,22.48 13.46,23.16 | v25.4,22.48 26.04,22.48 26.67,21.84 C3.1 26.67,14.61 27.94,13.34 BRA1.+
  Bottom 0.813: v18.41,22.48 v25.4,22.48
UNREG_12V  (via drill 0.5, 0.9)
  Top 0.762: v95.38,16.64 IC3.10
  Top 2.54: X2.2 28.87,5.42 24.13,10.16 BRA1.~@1 24.13,15.24 | 24.13,15.24 BRA1.~@2 | U$1.TIP 15.14,13.87 16.51,15.24 24.13,15.24
  Bottom 1.016: C2.+ 85.72,36.2
  Bottom 1.27: 98.81,36.2 98.81,20.07 v95.38,16.64
  Bottom 1.422: v31.11,33.66 31.11,35.56 30.48,36.2
  Bottom 1.778: 43.18,36.2 30.48,36.2 27.81,36.2 K1.1 | 73.66,36.2 58.42,36.2 | 58.42,36.2 43.18,36.2 | 43.18,36.2 43.18,39.88 K2.1 | K3.1 58.29,36.32 58.42,36.2 | 106.05,36.2 98.81,36.2 85.72,36.2 73.66,36.2 | 106.05,36.2 120.65,36.2 | 120.65,36.2 136.53,36.2 | 136.53,36.2 151.13,36.2 151.76,36.83 151.76,39.88 K8.1 | K7.1 136.4,36.32 136.53,36.2 | K6.1 121.16,36.7 120.65,36.2 | K5.1 105.92,36.32 106.05,36.2 | 73.66,36.2 73.66,39.88 K4.1 73.53,36.32 73.66,36.2 | v31.11,33.66 31.11,6.71 X2.2

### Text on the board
tNames: 1 | 8 | 4 | 5 | Bank 1 | A0 | A1 | A2 | Address | SC | I2C OUT | SCL | SDA | +5V | GND | 2016 ControlEverything.com | MCP23008 | SCR8xDPDT | REV.E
